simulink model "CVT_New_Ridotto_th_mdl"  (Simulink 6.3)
settings: Solver=ode45  StartTime=0.0  StopTime=10.0  RelTol=1e-3
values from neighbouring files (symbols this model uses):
  Tc = 0.05*ms    (= 5e-05)    [architetture_epicicloidale_statico.m]    (also in architetture_HEV_startstop_1.m; architetture_HEV_startstop_2.m; CVT_New.m; CVT_New_th.m)
  Wm_0 = 1*rpm    (= 0.10471975512)    [CVT_New.m]    (also in CVT_New_th.m)
libraries: simulink x1

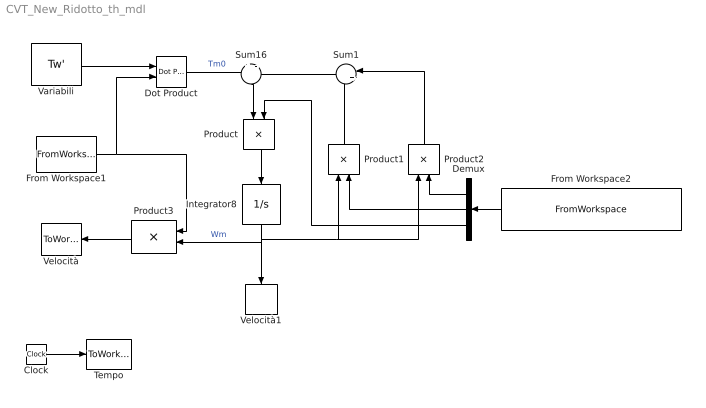
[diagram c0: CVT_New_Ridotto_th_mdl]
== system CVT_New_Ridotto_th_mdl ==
  Clock : Clock
  Demux : Demux  Orientation=left  Outputs=3
  Dot Product : simulink/Math Operations/Dot Product  InputSameDT=on  OutDataType=sfix(16)  OutScaling=2^-10  DoSatur=off
  From Workspace1 : FromWorkspace  VariableName=[time Tt_t]  SampleTime=0
  From Workspace2 : FromWorkspace  Orientation=left  VariableName=[time bt_th_t Jt_th_dot_t Jm1_th_t]  SampleTime=0
  Integrator8 : Integrator  Orientation=down  InitialCondition=Wm_0  LowerSaturationLimit=0
  Product : Product  Orientation=down
  Product1 : Product  Orientation=up
  Product2 : Product  Orientation=up
  Product3 : Product  Orientation=left  Multiplication=Matrix(*)
  Sum1 : Sum  Orientation=left  Inputs=|++
  Sum16 : Sum  Orientation=down  Inputs=+|-
  Tempo : ToWorkspace  VariableName=t  SampleTime=Tc  SaveFormat=Array
  Variabili : Constant  Value=Tw'
  Velocità : ToWorkspace  VariableName=Xt  SampleTime=Tc  SaveFormat=Array
  Velocità1 : ToWorkspace  VariableName=Wm  SampleTime=Tc  SaveFormat=Array
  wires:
  Clock/1 -> Tempo/1
  Dot Product/1 -> Sum16/1  "Tm0"
  Sum16/1 -> Product/1
  Integrator8/1 -> Velocità1/1, Product1/1, Product2/1, Product3/2  "Wm"
  Variabili/1 -> Dot Product/1
  Sum1/1 -> Sum16/2
  Product2/1 -> Sum1/1
  Product1/1 -> Sum1/2
  Product/1 -> Integrator8/1
  From Workspace2/1 -> Demux/1
  Demux/1 -> Product2/2
  Demux/2 -> Product1/2
  Demux/3 -> Product/2
  From Workspace1/1 -> Dot Product/2, Product3/1
  Product3/1 -> Velocità/1
